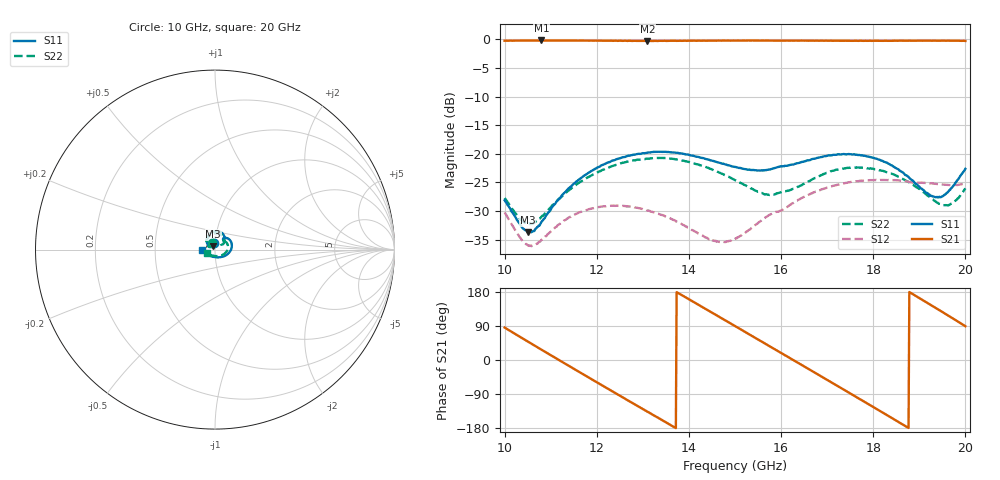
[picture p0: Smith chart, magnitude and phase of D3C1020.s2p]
! 11/5/2020 2:26:27 PM
! C:\USERS\DITOM\DESKTOP\SINGLE JUNCTION ISOLATOR DATA\10.0 - 20.0 GHZ (D3I1020).S2P
! CHANNEL.1
! TR.MEASUREMENT
! CORRECTED.DATA
# GHZ S RI R 50.0
! FREQ.GHZ  S11RE  S11IM  S21RE  S21IM  S12RE  S12IM  S22RE  S22IM
!; PortSelection: Port_12
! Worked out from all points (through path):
!   601 points, 10 GHz to 20 GHz, reference 50 ohm
!   highest |S21| = -0.20 dB at 10.8 GHz (marker M1); lowest = -0.3 dB at 13.1 GHz (marker M2)
!   lowest |S11| = -33.7 dB at 10.5 GHz (marker M3), VSWR 1.04, Z = 49 + j1.79 ohm
!   |S11| at or under -10 dB: start of sweep to end of sweep
!   |S22| runs from -32.3 to -20.7 dB; largest |S21 - S12| = 1
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10  -0.00418 0.0391  0.0744 0.9686  0.0158 -0.0265  -0.0179 0.0371
10.5  -0.00959 0.0182  0.6396 0.7352  0.00944 -0.0129  -0.0171 0.0177
10.8  -0.0203 0.0155  0.8687 0.4464  0.0133 -0.0119  -0.0249 0.0131
11.23333  -0.0362 0.023  0.9729 -0.0673  0.015 -0.0201  -0.038 0.0182
11.66667  -0.0456 0.0416  0.7983 -0.5591  0.00561 -0.0307  -0.0463 0.0343
12.38333  -0.0359 0.0804  0.0721 -0.9687  -0.0231 -0.0266  -0.0376 0.0699
13.1  -2.48e-05 0.1024  -0.6991 -0.6645  -0.032 0.00169  -0.00118 0.0908
13.35  0.0147 0.1033  -0.87 -0.4286  -0.028 0.0102  0.0144 0.091
14.1  0.047 0.0838  -0.8691 0.4377  -0.00963 0.0191  0.0483 0.0673
14.58333  0.0519 0.0676  -0.4729 0.8492  -0.00388 0.017  0.0527 0.0472
15  0.0501 0.0582  0.00653 0.9737  -0.00272 0.0179  0.0484 0.0337
15.41667  0.0459 0.0555  0.4871 0.8435  0.00206 0.0233  0.0397 0.0279
15.9  0.0455 0.061  0.8769 0.4226  0.0176 0.0257  0.0308 0.0329
16.28333  0.0511 0.0629  0.9717 -0.0237  0.0317 0.0202  0.0311 0.0388
16.66667  0.0616 0.0651  0.8529 -0.4682  0.0451 0.00267  0.0376 0.0462
17.11667  0.079 0.0573  0.4723 -0.8476  0.0439 -0.0287  0.0538 0.0466
17.51667  0.0909 0.0393  0.0101 -0.9707  0.0225 -0.0522  0.0668 0.0355
17.91667  0.0931 0.0134  -0.4567 -0.8566  -0.0106 -0.0579  0.0723 0.0172
18.35  0.0797 -0.0159  -0.8345 -0.4978  -0.0425 -0.041  0.068 -0.00535
19.1  0.0205 -0.0433  -0.8908 0.3917  -0.0541 0.0136  0.0312 -0.0339
19.58333  -0.0295 -0.034  -0.4937 0.8365  -0.0353 0.0405  -0.00738 -0.0349
20  -0.0739 -0.00342  0.0144 0.9669  -0.0161 0.053  -0.0463 -0.0189
